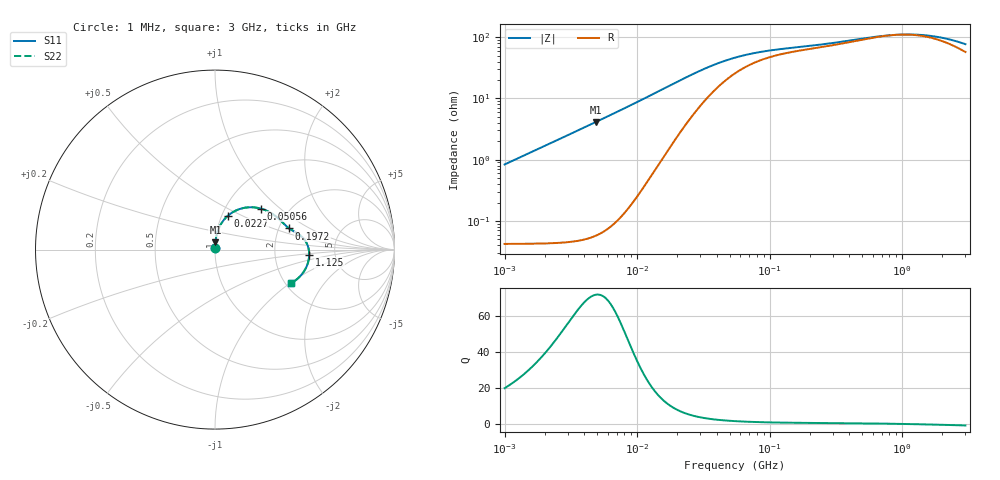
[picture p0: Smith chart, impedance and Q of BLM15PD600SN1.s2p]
! BLM15PD600SN1
# Hz S RI R 50
!Freq.(Hz) S11(Real) S11(Imag) S21(Real) S21(Imag) S12(Real) S12(Imag) S22(Real) S22(Imag)
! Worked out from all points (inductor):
!   401 points, 1 MHz to 3 GHz, reference 50 ohm
!   read as one part in series: L = 133 nH near 1.041 MHz
!   highest Q = 71.6 at 4.861 MHz (marker M1), where L = 134 nH
!   self-resonance near 927.7 MHz
!   S11 on the Smith chart (normalised r, x): 1 MHz: 1.00, +0.02; 22.7 MHz: 1.07, +0.42; 50.56 MHz: 1.45, +0.75; 197.2 MHz: 2.28, +0.66; 1.125 GHz: 3.19, -0.25; 3 GHz: 2.14, -1.02
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1000000  0.000491 0.00833  0.9995 -0.00833  0.9995 -0.00833  0.000491 0.00833
3823119  0.00152 0.0321  0.9985 -0.0321  0.9985 -0.0321  0.00152 0.0321
4861065  0.00225 0.0409  0.9978 -0.0409  0.9978 -0.0409  0.00225 0.0409
8861669  0.00755 0.0759  0.9924 -0.0759  0.9924 -0.0759  0.00755 0.0759
1.461624e7  0.025 0.127  0.975 -0.127  0.975 -0.127  0.025 0.127
2.270269e7  0.0719 0.1886  0.9281 -0.1886  0.9281 -0.1886  0.0719 0.1886
2.773354e7  0.1095 0.2143  0.8905 -0.2143  0.8905 -0.2143  0.1095 0.2143
3.387922e7  0.1562 0.2312  0.8438 -0.2312  0.8438 -0.2312  0.1562 0.2312
4.138676e7  0.2068 0.2359  0.7932 -0.2359  0.7932 -0.2359  0.2068 0.2359
5.055795e7  0.2549 0.2285  0.7451 -0.2285  0.7451 -0.2285  0.2549 0.2285
5.477226e7  0.2723 0.2229  0.7277 -0.2229  0.7277 -0.2229  0.2723 0.2229
7.105049e7  0.3199 0.1989  0.6801 -0.1989  0.6801 -0.1989  0.3199 0.1989
9.216659e7  0.354 0.1725  0.646 -0.1725  0.646 -0.1725  0.354 0.1725
1.971969e8  0.4131 0.118  0.5869 -0.118  0.5869 -0.118  0.4131 0.118
2.094008e8  0.417 0.1153  0.583 -0.1153  0.583 -0.1153  0.417 0.1153
4.480278e8  0.4764 0.0783  0.5236 -0.0783  0.5236 -0.0783  0.4764 0.0783
8.005644e8  0.5172 0.02  0.4828 -0.02  0.4828 -0.02  0.5172 0.02
1.125055e9  0.525 -0.0287  0.475 0.0287  0.475 0.0287  0.525 -0.0287
1.45942e9  0.5188 -0.0707  0.4812 0.0707  0.4812 0.0707  0.5188 -0.0707
1.855641e9  0.5017 -0.1115  0.4983 0.1115  0.4983 0.1115  0.5017 -0.1115
2.312676e9  0.4743 -0.1485  0.5257 0.1485  0.5257 0.1485  0.4743 -0.1485
3e9  0.4248 -0.1872  0.5752 0.1872  0.5752 0.1872  0.4248 -0.1872
